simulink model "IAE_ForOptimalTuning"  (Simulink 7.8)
settings: Solver=ode3  StartTime=0.0  StopTime=100  FixedStep=0.01  RelTol=1e-6
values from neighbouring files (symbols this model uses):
  delay = delayv(i)    [example.m]    (also in IAE_Simulink.m; Robustness_SP.m; Robustness_SP_P.m; Robustness_SP_PI.m)
libraries: simulink x2

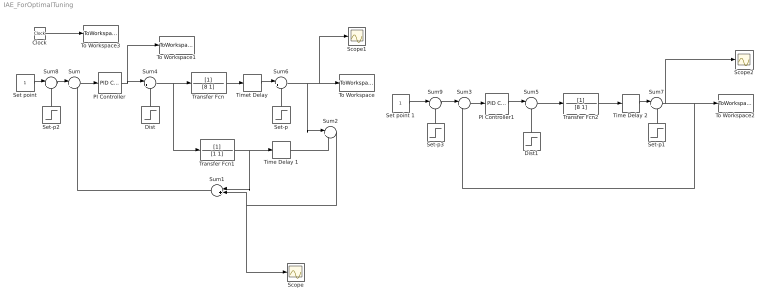
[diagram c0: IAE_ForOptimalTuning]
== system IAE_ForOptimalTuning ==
  Clock : Clock
  Dist : Step  Time=20  SampleTime=0
  Dist1 : Step  Time=20  SampleTime=0
  PI Controller : simulink/Continuous/PID Controller  Controller=PI  TimeDomain=Continuous-time  SampleTime=1  IntegratorMethod=Forward Euler  FilterMethod=Forward Euler  Form=Ideal  P=1.70  I=0.73  D=0  N=100  InitialConditionSource=internal  InitialConditionForIntegrator=0  InitialConditionForFilter=0  ExternalReset=none  LimitOutput=off  UpperSaturationLimit=inf  LowerSaturationLimit=-inf  LinearizeAsGain=off  AntiWindupMode=none  Kb=1  TrackingMode=off  Kt=1  PParamMin=[]  PParamMax=[]  IParamMin=[]  IParamMax=[]  DParamMin=[]  DParamMax=[]  NParamMin=[]  NParamMax=[]  KbParamMin=[]  KbParamMax=[]  KtParamMin=[]  KtParamMax=[]  POutMin=[]  POutMax=[]  IOutMin=[]  IOutMax=[]  DOutMin=[]  DOutMax=[]  NOutMin=[]  NOutMax=[]  KbOutMin=[]  KbOutMax=[]  KtOutMin=[]  KtOutMax=[]  IntegratorOutMin=[]  IntegratorOutMax=[]  FilterOutMin=[]  FilterOutMax=[]  SumOutMin=[]  SumOutMax=[]  SumI1OutMin=[]  SumI1OutMax=[]  SumI2OutMin=[]  SumI2OutMax=[]  SumI3OutMin=[]  SumI3OutMax=[]  SumDOutMin=[]  SumDOutMax=[]  SaturationOutMin=[]  SaturationOutMax=[]  IntegratorContinuousStateAttributes=''  IntegratorStateMustResolveToSignalObject=off  IntegratorRTWStateStorageClass=Auto  FilterContinuousStateAttributes=''  FilterStateMustResolveToSignalObject=off  FilterRTWStateStorageClass=Auto
  PI Controller1 : simulink/Continuous/PID Controller  Controller=PI  TimeDomain=Continuous-time  SampleTime=1  IntegratorMethod=Forward Euler  FilterMethod=Forward Euler  Form=Ideal  P=2.83  I=0.39  D=0  N=100  InitialConditionSource=internal  InitialConditionForIntegrator=0  InitialConditionForFilter=0  ExternalReset=none  LimitOutput=off  UpperSaturationLimit=inf  LowerSaturationLimit=-inf  LinearizeAsGain=off  AntiWindupMode=none  Kb=1  TrackingMode=off  Kt=1  PParamMin=[]  PParamMax=[]  IParamMin=[]  IParamMax=[]  DParamMin=[]  DParamMax=[]  NParamMin=[]  NParamMax=[]  KbParamMin=[]  KbParamMax=[]  KtParamMin=[]  KtParamMax=[]  POutMin=[]  POutMax=[]  IOutMin=[]  IOutMax=[]  DOutMin=[]  DOutMax=[]  NOutMin=[]  NOutMax=[]  KbOutMin=[]  KbOutMax=[]  KtOutMin=[]  KtOutMax=[]  IntegratorOutMin=[]  IntegratorOutMax=[]  FilterOutMin=[]  FilterOutMax=[]  SumOutMin=[]  SumOutMax=[]  SumI1OutMin=[]  SumI1OutMax=[]  SumI2OutMin=[]  SumI2OutMax=[]  SumI3OutMin=[]  SumI3OutMax=[]  SumDOutMin=[]  SumDOutMax=[]  SaturationOutMin=[]  SaturationOutMax=[]  IntegratorContinuousStateAttributes=''  IntegratorStateMustResolveToSignalObject=off  IntegratorRTWStateStorageClass=Auto  FilterContinuousStateAttributes=''  FilterStateMustResolveToSignalObject=off  FilterRTWStateStorageClass=Auto
  Scope : Scope
  Scope1 : Scope
  Scope2 : Scope
  Set point : Constant
  Set point 1 : Constant
  Set-p : Step  Time=0  SampleTime=0
  Set-p1 : Step  Time=0  SampleTime=0
  Set-p2 : Step  Time=0  After=0  SampleTime=0
  Set-p3 : Step  Time=0  After=0  SampleTime=0
  Sum{,2..3,8..9} (5 alike) : Sum  Inputs=|+-
  Sum{1,4..7} (5 alike) : Sum  Inputs=|++
  Time Delay 1 : TransportDelay
  Time Delay 2 : TransportDelay  DelayTime=delay
  Timet Delay : TransportDelay  DelayTime=delay
  To Workspace : ToWorkspace  VariableName=Ysp  SampleTime=-1  SaveFormat=Array
  To Workspace1 : ToWorkspace  VariableName=usp  SampleTime=-1  SaveFormat=Structure
  To Workspace2 : ToWorkspace  VariableName=Ypi  SampleTime=-1  SaveFormat=Array
  To Workspace3 : ToWorkspace  VariableName=time  SampleTime=-1  SaveFormat=Array
  Transfer Fcn : TransferFcn  Denominator=[8 1]
  Transfer Fcn1 : TransferFcn  Denominator=[1 1]
  Transfer Fcn2 : TransferFcn  Denominator=[8 1]
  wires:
  Sum/1 -> PI Controller/1
  PI Controller/1 -> To Workspace1/1, Sum4/1
  Transfer Fcn/1 -> Timet Delay/1
  Transfer Fcn1/1 -> Time Delay 1/1, Sum1/1
  Time Delay 1/1 -> Sum2/2
  Sum2/1 -> Sum1/2, Scope/1
  Sum1/1 -> Sum/2
  Transfer Fcn2/1 -> Time Delay 2/1
  Sum3/1 -> PI Controller1/1
  Clock/1 -> To Workspace3/1
  Sum4/1 -> Transfer Fcn/1, Transfer Fcn1/1
  PI Controller1/1 -> Sum5/1
  Sum5/1 -> Transfer Fcn2/1
  Timet Delay/1 -> Sum6/1
  Sum6/1 -> To Workspace/1, Scope1/1, Sum2/1
  Time Delay 2/1 -> Sum7/1
  Sum7/1 -> Scope2/1, To Workspace2/1, Sum3/2
  Dist/1 -> Sum4/2
  Set-p/1 -> Sum6/2
  Dist1/1 -> Sum5/2
  Set-p1/1 -> Sum7/2
  Set point/1 -> Sum8/1
  Sum8/1 -> Sum/1
  Set-p2/1 -> Sum8/2
  Set point 1/1 -> Sum9/1
  Sum9/1 -> Sum3/1
  Set-p3/1 -> Sum9/2
